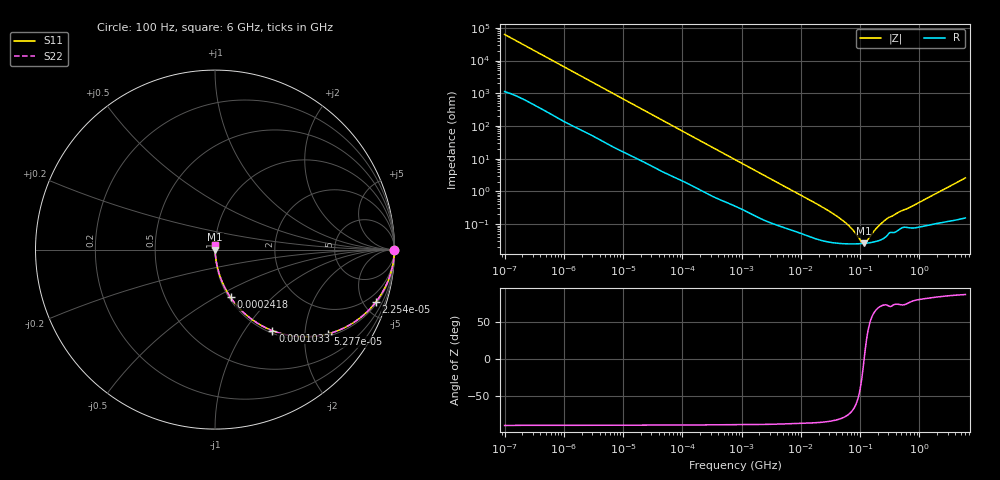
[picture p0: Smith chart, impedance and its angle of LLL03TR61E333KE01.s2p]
!Murata Part Number: LLL03TR61E333KE01
!These Parameters are Measured in Series Mode Connection
!Data Generated on Mar 13, 2026
!  o--ll--o
!Port1  Port2
!  o------o
!Operation Temp=25[degC], DC Bias Voltage=0[V]
!Freq. Start=100[Hz] Stop=6[GHz] 401[Steps]
# Hz S RI R 50
!Freq.(Hz) S11(Real) S11(Imag) S21(Real) S21(Imag) S12(Real) S12(Imag) S22(Real) S22(Imag)
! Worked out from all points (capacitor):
!   401 points, 100 Hz to 6 GHz, reference 50 ohm
!   read as one part in series: C = 25.2 nF near 109 Hz
!   lowest |Z| = 25.6 mohm at 116.7 MHz (marker M1)
!   series resonance near 117.1 MHz, so ESL is about 73 pH
!   S11 on the Smith chart (normalised r, x): 100 Hz: open; 22.54 kHz: 1.16, -6.05; 52.77 kHz: 1.07, -2.62; 103.3 kHz: 1.04, -1.35; 241.8 kHz: 1.02, -0.59; 6 GHz: 1.00, +0.05
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100  1 -0.00159  3.1e-05 0.00159  3.1e-05 0.00159  1 -0.00159
2008  0.9984 -0.0305  0.00162 0.0305  0.00162 0.0305  0.9984 -0.0305
7695  0.9844 -0.1127  0.0156 0.1127  0.0156 0.1127  0.9844 -0.1127
22537  0.8954 -0.2933  0.1046 0.2933  0.1046 0.2933  0.8954 -0.2933
40335  0.7388 -0.4262  0.2612 0.4262  0.2612 0.4262  0.7388 -0.4262
52766  0.6284 -0.4698  0.3716 0.4698  0.3716 0.4698  0.6284 -0.4698
72189  0.4814 -0.4856  0.5186 0.4856  0.5186 0.4856  0.4814 -0.4856
103284  0.3195 -0.4515  0.6805 0.4515  0.6805 0.4515  0.3195 -0.4515
154540  0.1799 -0.369  0.8201 0.369  0.8201 0.369  0.1799 -0.369
241822  0.0866 -0.2662  0.9134 0.2662  0.9134 0.2662  0.0866 -0.2662
774597  0.0122 -0.0925  0.9878 0.0925  0.9878 0.0925  0.0122 -0.0925
2481164  0.00218 -0.03  0.9978 0.03  0.9978 0.03  0.00218 -0.03
1.555665e7  0.00041 -0.00496  0.9996 0.00496  0.9996 0.00496  0.00041 -0.00496
3.184506e7  0.000281 -0.00231  0.9997 0.00231  0.9997 0.00231  0.000281 -0.00231
5.211241e7  0.000253 -0.00123  0.9997 0.00123  0.9997 0.00123  0.000253 -0.00123
7.455971e7  0.000248 -0.000637  0.9998 0.000637  0.9998 0.000637  0.000248 -0.000637
1.066761e8  0.000253 -0.000128  0.9997 0.000128  0.9997 0.000128  0.000253 -0.000128
1.166697e8  0.000256 -5.3e-06  0.9997 5.3e-06  0.9997 5.3e-06  0.000256 -5.3e-06
1.334425e8  0.000263 0.000179  0.9997 -0.000179  0.9997 -0.000179  0.000263 0.000179
2.088084e8  0.000314 0.00084  0.9997 -0.00084  0.9997 -0.00084  0.000314 0.00084
3.124326e8  0.000537 0.00154  0.9995 -0.00154  0.9995 -0.00154  0.000537 0.00154
6e9  0.0022 0.0257  0.9978 -0.0257  0.9978 -0.0257  0.0022 0.0257
